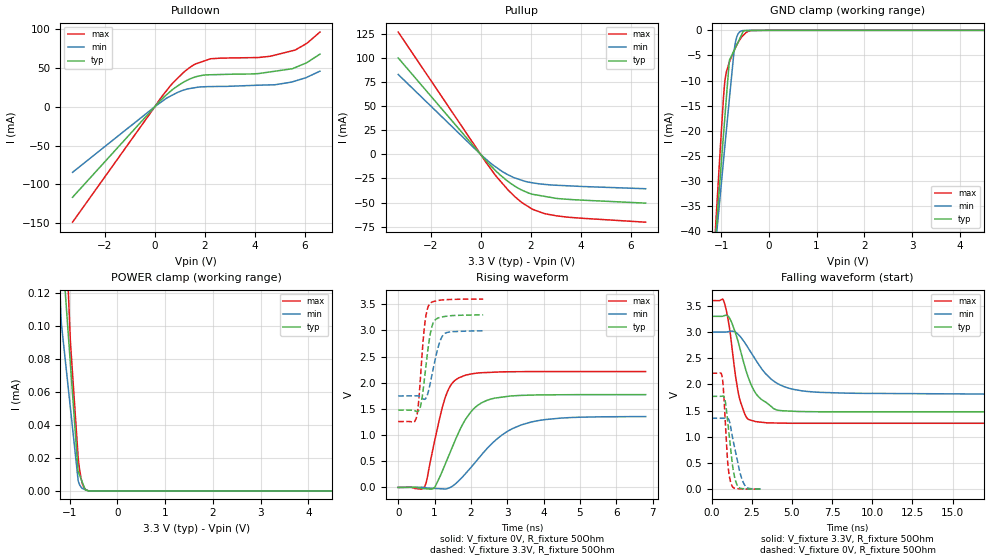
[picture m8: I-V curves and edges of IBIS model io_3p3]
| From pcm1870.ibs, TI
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|   io_3p3 Model
[Model]   io_3p3
Model_type   I/O
Polarity   Non-Inverting
Enable   Active-Low
Vinl = 0.99
Vinh = 2.31
Vmeas = 1.65
Vref = 1.65
Cref = 400pF
Rref = 50
|   typ   min   max
C_comp   1.899e-12   1.797e-12   1.961e-12
[Model spec]
Vinl   0.99   0.9   1.08
Vinh   2.31   2.1   2.52
| Where nom  PVT is Nominal Process, 3.3V, 26C
|   Fast PVT is Strong Process,  3.6V, -40C
|   Slow PVT is Weak Process,   3V, 86C
[Voltage Range]   3.3   3   3.6
|Ambient Temperature   25   85   -40
|Junction Temperature
[Temperature Range]   26   86   -40
[Pullup Reference]   3.3   3   3.6
[Pulldown Reference]   0   0   0
[Power Clamp Reference]   3.3   3   3.6
[GND Clamp Reference]   0   0   0
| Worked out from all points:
|   slope of the pulldown table from 0 to 0.495 V, typ, clamps not added: 30.8 ohm
|   slope of the pullup table from 0 to 0.495 V, typ, clamps not added: 34.8 ohm
|   GND clamp passes 1 mA (typ) near -0.58 V on its own axis
|   POWER clamp passes 1 mA (typ) near -2.20 V on its own axis
|   falling waveform, V_fixture 3.3V, R_fixture 50Ohm: 20-80 % time 1.19ns typ, 2.06ns min, 657ps max; typ from 3.3 V to 1.48 V
|   rising waveform, V_fixture 0V, R_fixture 50Ohm: 20-80 % time 733ps typ, 1.18ns min, 453ps max; typ from 0 V to 1.77 V
|   rising waveform, V_fixture 3.3V, R_fixture 50Ohm: 20-80 % time 201ps typ, 244ps min, 159ps max; typ from 1.48 V to 3.29 V
|   falling waveform, V_fixture 0V, R_fixture 50Ohm: 20-80 % time 395ps typ, 561ps min, 260ps max; typ from 1.77 V to 0.002 V
[Pulldown]
|   Voltage   I(typ)   I(min)   I(max)
-3.3V     -116.5mA   -84.42mA   -148.5mA
204.6mV   7.28mA     4.831mA    9.794mA
714mV     22.1mA     15.03mA    30.35mA
1.355V    34.85mA    23mA       49.31mA
1.589V    37.79mA    24.19mA    54.3mA
1.917V    40.26mA    25.39mA    57.97mA
2.222V    40.84mA    25.67mA    61.38mA
4.138V    42.37mA    27.44mA    62.98mA
4.797V    45.4mA     27.99mA    66.02mA
5.606V    50.05mA    32.81mA    72.53mA
6.082V    56.53mA    37.7mA     81.29mA
6.6V      67.25mA    45.42mA    95.62mA
[GND Clamp]
|   Voltage   I(typ)   I(min)   I(max)
-3.3V     -316.9mA   -268mA     -391.9mA
-1.115V   -41.24mA   -42.61mA   -38.94mA
-1.021V   -29.54mA   -33.14mA   -24.12mA
-949.2mV  -20.65mA   -25.85mA   -13.18mA
-906mV    -15.4mA    -21.5mA    -9.078mA
-825mV    -5.93mA    -13.45mA   -6.269mA
-720mV    -3.842mA   -3.574mA   -3.911mA
-648mV    -2.41mA    -753.9uA   -2.497mA
-567mV    -799uA     -93.36uA   -1.3mA
-534.6mV  -154.6uA   -39.82uA   -983.6uA
-373.2mV  -37.21uA   -260.9nA   -41.52uA
6.6V      0A         0A         0A
[Pullup]
|   Voltage   I(typ)   I(min)   I(max)
-3.3V     100.2mA    83.06mA    127.1mA
3mV       -189.6uA   -162uA     -246.2uA
363mV     -10.78mA   -8.423mA   -13.7mA
638.4mV   -18mA      -13.71mA   -23.32mA
1.103V    -28.27mA   -21.31mA   -37.21mA
1.643V    -37.09mA   -26.87mA   -49.95mA
2.064V    -41.39mA   -29.49mA   -56.97mA
2.525V    -43.47mA   -31.07mA   -61.32mA
3.018V    -45.7mA    -32.05mA   -63.8mA
3.983V    -47.45mA   -33.24mA   -66.26mA
6.6V      -50.64mA   -35.68mA   -70.46mA
[POWER Clamp]
|   Voltage   I(typ)   I(min)   I(max)
-3.3V     2.454mA    1.841mA    2.082mA
-2.086V   842.8uA    859.9uA    936.3uA
-1.185V   157.5uA    106.8uA    231.2uA
-1.169V   151.1uA    99.86uA    219.1uA
-985.2mV  76.84uA    50.18uA    90.22uA
-822mV    11.82uA    6.025uA    20.04uA
-783.6mV  8.89uA     3.22uA     11.01uA
-762mV    7.243uA    2.349uA    7.554uA
-726mV    4.499uA    1.448uA    3.681uA
-675.6mV  715.3nA    706.4nA    1.109uA
-603.6mV  0A         0A         0A
6.6V      0A         0A         0A
[Ramp]
R_load = 50
|   typ   min   max
dV/dt_r   1.06379/7.30313e-10   0.812601/1.17719e-09   1.32828/4.52991e-10
dV/dt_f   1.09414/1.19212e-09   0.751806/2.05343e-09   1.40532/6.56875e-10
[Falling Waveform]
V_fixture = 3.3V
V_fixture_min = 3V
V_fixture_max = 3.6V
R_fixture = 50Ohm
|   Time   V(typ)   V(min)   V(max)
0s        3.3V       3V         3.6V
765.1ps   3.309V     3V         3.586V
1.174ns   3.234V     3.015V     2.947V
1.507ns   2.964V     2.995V     2.129V
1.77ns    2.682V     2.92V      1.695V
2.151ns   2.257V     2.757V     1.381V
2.695ns   1.857V     2.494V     1.294V
4.024ns   1.517V     2.032V     1.263V
5.974ns   1.481V     1.865V     1.259V
30ns      1.476V     1.747V     1.258V
[Rising Waveform]
V_fixture = 0V
V_fixture_min = 0V
V_fixture_max = 0V
R_fixture = 50Ohm
|   Time   V(typ)   V(min)   V(max)
0s        476.9pV    717.9pV    417.6pV
734.3ps   -24.42mV   -3.603mV   29.01mV
1.015ns   15mV       -19.8mV    932.5mV
1.277ns   417.2mV    -29.42mV   1.68V
1.436ns   683.1mV    2.373mV    1.941V
1.664ns   1.052V     127.5mV    2.092V
1.995ns   1.44V      376.7mV    2.166V
2.301ns   1.619V     629.8mV    2.191V
3.377ns   1.758V     1.192V     2.211V
6.809ns   1.772V     1.354V     2.213V
[Rising Waveform]
V_fixture = 3.3V
V_fixture_min = 3V
V_fixture_max = 3.6V
R_fixture = 50Ohm
|   Time   V(typ)   V(min)   V(max)
0s        1.476V     1.747V     1.258V
500.6ps   1.451V     1.75V      1.335V
554.5ps   1.459V     1.747V     1.58V
619.4ps   1.566V     1.724V     2.177V
734.3ps   2.149V     1.685V     3.147V
855.6ps   2.822V     1.911V     3.494V
985.2ps   3.174V     2.341V     3.553V
1.141ns   3.245V     2.775V     3.575V
1.249ns   3.262V     2.922V     3.582V
2.338ns   3.295V     2.992V     3.597V
[Falling Waveform]
V_fixture = 0V
V_fixture_min = 0V
V_fixture_max = 0V
R_fixture = 50Ohm
|   Time   V(typ)   V(min)   V(max)
0s        1.773V     1.354V     2.214V
656.7ps   1.776V     1.354V     2.154V
734.3ps   1.775V     1.354V     1.918V
839ps     1.703V     1.357V     1.37V
1.01ns    1.273V     1.354V     492.2mV
1.131ns   931.6mV    1.27V      210.1mV
1.261ns   570.1mV    1.061V     70.68mV
1.546ns   112.7mV    634.5mV    12.17mV
2.02ns    9.4mV      100.1mV    3.326mV
3.063ns   1.766mV    2.709mV    710.9uV
